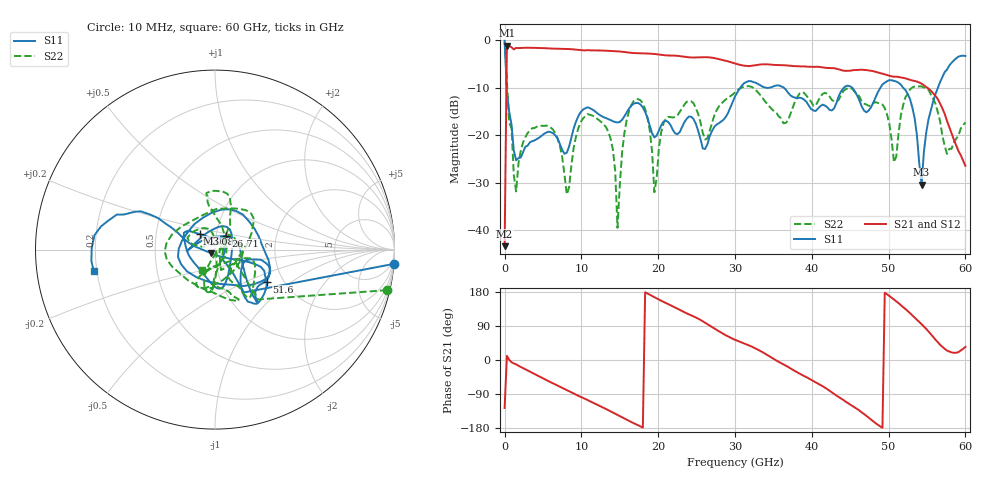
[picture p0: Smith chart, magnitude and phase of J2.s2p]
!Keysight Technologies,N5227A,US51270214,A.10.65.11
!Date: Thursday, October 15, 2020 08:19:49
!Correction: S11(Full 2 Port(1,2))
!S21(Full 2 Port(1,2))
!S12(Full 2 Port(1,2))
!S22(Full 2 Port(1,2))
!S2P File: Measurements: S11, S21, S12, S22:
# Hz S  dB  R 50
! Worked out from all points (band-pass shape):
!   201 points, 10 MHz to 60 GHz, reference 50 ohm
!   highest |S21| = -1.12 dB at 309.9 MHz (marker M1); lowest = -43.4 dB at 10 MHz (marker M2)
!   |S21| within 3 dB of the highest: 288.7 MHz to 28.4 GHz (28.11 GHz wide, 196 % of centre)
!   lowest |S11| = -30.4 dB at 54.3 GHz (marker M3), VSWR 1.06, Z = 47.7 - j1.89 ohm
!   |S11| at or under -10 dB: 287.5 MHz to 30.69 GHz (30.4 GHz wide, 196 % of centre); 36.38 GHz to 44.18 GHz (7.795 GHz wide, 19.4 % of centre); 51.9 GHz to 56.41 GHz (4.509 GHz wide, 8.33 % of centre)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
!   |S22| runs from -39.5 to -0.1 dB; largest |S21 - S12| = 0.14
!   S11 on the Smith chart (normalised r, x): 10 MHz: -0, -25; 9.008 GHz: 0.84, +0.15; 26.71 GHz: 1.12, +0.17; 51.6 GHz: 1.64, -0.67; 60 GHz: 0.19, -0.09
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1e7  0.00 -4.6  -43.42 -126.6  -46.51 -130.0  -0.13 -13.3
3.0995e8  -10.81 -56.0  -1.12 11.0  -1.85 19.1  -8.71 -49.3
1.50975e9  -25.29 -16.7  -1.57 -11.4  -1.39 -10.2  -31.86 2.3
3.6094e9  -21.25 39.2  -1.54 -34.1  -1.49 -34.1  -18.52 40.6
8.10865e9  -23.68 98.0  -1.79 -79.3  -1.79 -79.5  -32.51 82.4
9.0085e9  -18.55 133.7  -1.89 -88.6  -1.89 -88.6  -22.59 167.6
1.02083e10  -14.60 146.5  -2.08 -100.0  -2.06 -100.1  -16.48 164.0
1.38077e10  -16.81 -161.1  -2.21 -135.5  -2.22 -135.5  -20.72 98.6
1.470755e10  -17.31 -139.0  -2.29 -144.8  -2.31 -144.9  -39.53 62.8
1.650725e10  -13.77 -91.3  -2.62 -163.7  -2.64 -163.7  -13.65 -92.4
1.86069e10  -16.37 -60.4  -2.75 175.5  -2.77 175.5  -16.30 -111.6
1.950675e10  -20.46 -9.7  -2.85 165.5  -2.87 165.4  -32.02 -84.3
2.010665e10  -19.00 31.8  -2.97 159.2  -2.98 159.2  -22.51 19.6
2.670555e10  -20.22 51.6  -3.57 90.8  -3.61 90.8  -19.08 -34.0
3.0005e10  -11.83 -45.2  -4.86 53.3  -4.90 53.2  -10.95 -39.9
4.02033e10  -14.77 129.0  -5.55 -55.6  -5.57 -55.8  -13.77 107.1
5.010165e10  -8.36 -52.1  -7.44 168.8  -7.46 169.3  -17.67 -87.5
5.16014e10  -9.34 -32.0  -7.82 144.6  -7.82 144.3  -15.78 58.9
5.430095e10  -30.43 -138.8  -9.13 94.4  -9.14 94.3  -9.71 93.5
5.610065e10  -11.34 153.2  -11.69 53.6  -11.74 54.0  -13.35 93.6
5.76004e10  -6.16 154.6  -16.96 24.9  -16.92 25.1  -23.93 -4.3
6e10  -3.28 -169.9  -26.46 34.5  -26.54 34.6  -17.27 -123.3
